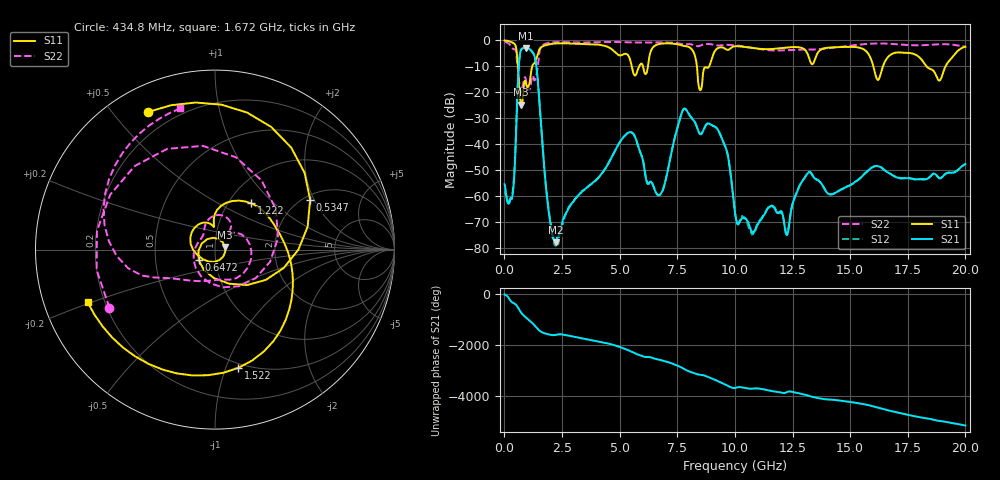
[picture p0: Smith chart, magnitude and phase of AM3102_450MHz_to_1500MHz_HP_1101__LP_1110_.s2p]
!Agilent Technologies,E8364B,MY43040894,A.07.50.67
!Agilent E8364B: A.07.50.67
!Date: Thursday, January 11, 2018 06:41:01
!Correction: S11(Full 2 Port(1,2))
!S21(Full 2 Port(1,2))
!S12(Full 2 Port(1,2))
!S22(Full 2 Port(1,2))
!S2P File: Measurements: S11, S21, S12, S22:
# Hz S  dB  R 50
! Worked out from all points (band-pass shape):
!   1601 points, 10 MHz to 20 GHz, reference 50 ohm
!   highest |S21| = -2.98 dB at 922 MHz (marker M1); lowest = -77.7 dB at 2.234 GHz (marker M2)
!   |S21| within 3 dB of the highest: 666.3 MHz to 1.304 GHz (638.1 MHz wide, 64.8 % of centre)
!   lowest |S11| = -24.7 dB at 734.6 MHz (marker M3), VSWR 1.12, Z = 55.9 + j1.61 ohm
!   |S11| at or under -10 dB: 587.2 MHz to 1.209 GHz (621.8 MHz wide, 69.2 % of centre); 8.352 GHz to 8.885 GHz (533.2 MHz wide, 6.19 % of centre); 18.31 GHz to 19.14 GHz (828.2 MHz wide, 4.42 % of centre)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
!   |S22| runs from -20.1 to -0.5 dB; largest |S21 - S12| = 0.0011
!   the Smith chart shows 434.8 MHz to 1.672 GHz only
!   S11 on the Smith chart (normalised r, x): 434.8 MHz: 0.11, +0.62; 534.7 MHz: 2.17, +1.86; 647.2 MHz: 0.83, -0.10; 1.222 GHz: 1.27, +0.73; 1.522 GHz: 0.46, -1.11; 1.672 GHz: 0.14, -0.20
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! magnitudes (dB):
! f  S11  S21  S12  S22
! 10 MHz  -0.1  -55.3  -58.5  -0.5
! 434.8 MHz  -1.4  -51.0  -50.3  -3.5
! 534.7 MHz  -4.5  -27.7  -27.8  -6.7
! 647.2 MHz  -19.4  -7.6  -7.6  -16.5
! 734.6 MHz  -24.7  -3.5  -3.5  -19.8
! 922 MHz  -16.0  -3.0  -3.0  -14.6
! 1.222 GHz  -9.7  -4.6  -4.6  -13.6
! 1.522 GHz  -3.5  -24.1  -24.1  -4.5
! 1.672 GHz  -2.3  -42.7  -42.8  -1.8
! 2.234 GHz  -1.2  -77.7  -78.9  -0.7
! 3.346 GHz  -1.4  -58.3  -58.3  -0.9
! 5.457 GHz  -7.5  -35.3  -35.3  -0.8
! 6.682 GHz  -1.5  -59.5  -59.6  -0.8
! 7.831 GHz  -2.2  -26.3  -26.3  -1.6
! 8.493 GHz  -19.2  -36.0  -36.1  -2.1
! 9.318 GHz  -2.8  -35.3  -35.3  -2.0
! 10.01 GHz  -2.3  -66.3  -66.2  -1.9
! 12.27 GHz  -2.8  -74.8  -74.0  -3.8
! 13.34 GHz  -9.2  -51.5  -51.5  -3.6
! 16.68 GHz  -6.1  -51.0  -51.0  -1.3
! 18.86 GHz  -15.5  -53.0  -52.9  -1.5
! 20 GHz  -2.5  -47.6  -47.6  -2.4
